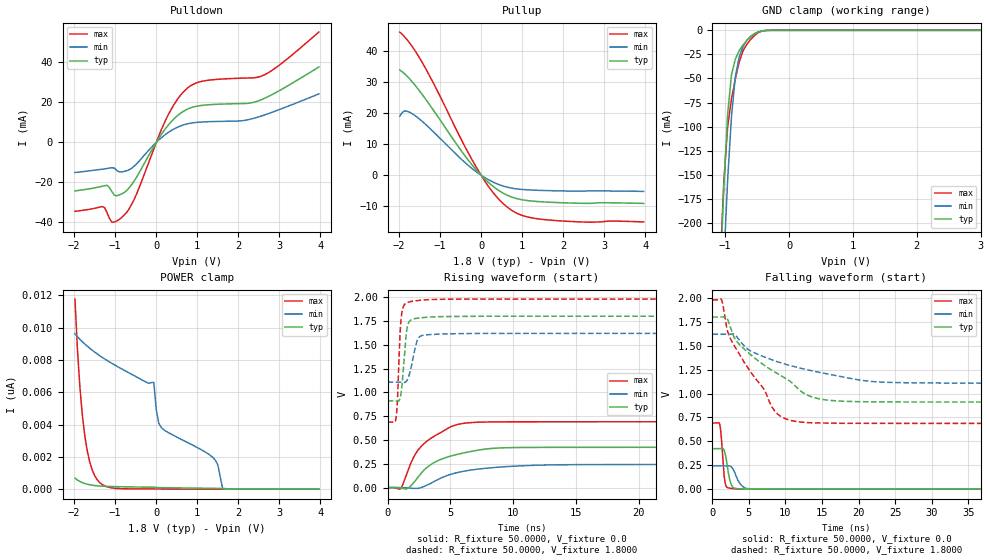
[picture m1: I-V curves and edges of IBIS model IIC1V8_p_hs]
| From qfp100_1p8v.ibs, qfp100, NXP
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[Model] IIC1V8_p_hs
|   Model IIC1V8_p_hs
| This model was characterised for following simulation conditions:
| External (pad) voltage:
|   - Typ: 1.8V,   - Min: 1.62V,   - Max: 1.98V
| Library cells for typ/min/max conditions are connected as defined below:
|  IO - External Pad
|  A - Core Input
|  EN - Output Buffer Enable
|  BOOST - vdde
|  EGP - vdd
|  EHS - vdd
|  ENZI - vdd
|  EPD - gnd
|  EPUN - vdd
|  ZI - NC
|  ZIF - NC
|  gnd - gnd
|  gnde - gnde
|  vdd - vdd
|  vdde - vdde
| All other pins connected to ground
Model_type I/O
Polarity   Non-Inverting
Enable   Active-Low
Vinl =   0.5400V
Vinh =   1.2600V
Vmeas =  0.9000V
Cref =   0.0F
Rref =   1.0000k
Vref =   0.0V
C_comp   3.6452pF   3.5037pF   3.7805pF
|C_comp_pullup   0.9522pF   0.9264pF   0.9623pF
|C_comp_pulldown   2.3410pF   2.4925pF   2.1970pF
[Model Spec]
| variable   typ   min   max
Vinh   0.5400V   0.4860V   0.5940V
Vinl   1.2600V   1.1340V   1.3860V
Vmeas   0.9000V   0.8100V   0.9900V
[Temperature Range]   25.0000   0.1250k   -40.0000
[Voltage Range]   1.8000V   1.6200V   1.9800V
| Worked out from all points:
|   slope of the pulldown table from 0 to 0.27 V, typ, clamps not added: 33.4 ohm
|   slope of the pullup table from 0 to 0.27 V, typ, clamps not added: 80.7 ohm
|   GND clamp passes 1 mA (typ) near -0.44 V on its own axis
|   rising waveform, R_fixture 50.0000, V_fixture 0.0: 20-80 % time 2.95ns typ, 3.71ns min, 2.38ns max; typ from 0 V to 0.423 V
|   rising waveform, R_fixture 50.0000, V_fixture 1.8000: 20-80 % time 334ps typ, 515ps min, 244ps max; typ from 0.911 V to 1.8 V
|   falling waveform, R_fixture 50.0000, V_fixture 0.0: 20-80 % time 582ps typ, 939ps min, 400ps max; typ from 0.423 V to 0 V
|   falling waveform, R_fixture 50.0000, V_fixture 1.8000: 20-80 % time 8.42ns typ, 11.2ns min, 5.75ns max; typ from 1.8 V to 0.911 V
[Pulldown]
|Voltage   I(typ)   I(min)   I(max)
-1.98V    -24.22mA   -15.04mA   -34.42mA
-1.32V    -21.94mA   -13.41mA   -32.06mA
-1.2V     -21.45mA   -13.05mA   -35.06mA
-1.08V    -24.63mA   -12.6mA    -39.9mA
-900mV    -26.23mA   -14.78mA   -38.53mA
-720mV    -24.07mA   -14.13mA   -34.99mA
-540mV    -19.33mA   -11.9mA    -28.53mA
300mV     8.856mA    5.096mA    14.12mA
720mV     16.26mA    9.117mA    26.48mA
1.14V     18.6mA     10.26mA    30.69mA
2.58V     21.56mA    13.35mA    33.32mA
3.96V     37.73mA    24.28mA    55.2mA
[Pullup]
|Voltage   I(typ)   I(min)   I(max)
-1.98V    33.84mA    18.97mA    46mA
-1.86V    32.57mA    20.67mA    44.44mA
-1.62V    29.12mA    19.27mA    40.26mA
-1.2V     21.64mA    14.46mA    30.6mA
-420mV    6.732mA    4.415mA    9.888mA
0V        251.1fA    74.01pA    -178.6fA
360mV     -4.265mA   -2.608mA   -6.666mA
660mV     -6.57mA    -3.917mA   -10.5mA
1.02V     -7.945mA   -4.606mA   -13.01mA
1.56V     -8.618mA   -4.934mA   -14.29mA
2.64V     -9.058mA   -5.064mA   -15.11mA
3.96V     -9.081mA   -5.209mA   -15.04mA
[GND_clamp]
|Voltage   I(typ)   I(min)   I(max)
-1.98V    -2.104A    -2.075A    -2.136A
-1.08V    -259.3mA   -333mA     -246.9mA
-1.02V    -161.8mA   -238.7mA   -157.1mA
-960mV    -86.74mA   -154.7mA   -99.46mA
-900mV    -45.95mA   -88.82mA   -71.05mA
-840mV    -29.9mA    -47.99mA   -50.25mA
-780mV    -21.15mA   -27.64mA   -32.98mA
-720mV    -15.16mA   -16.87mA   -21.26mA
-660mV    -10.56mA   -10.24mA   -14.56mA
-540mV    -3.788mA   -3.398mA   -5.292mA
-300mV    -15.94uA   -36uA      -16.34uA
3.96V     0A         0A         0A
[POWER_clamp]
|Voltage   I(typ)   I(min)   I(max)
-1.98V    679.6pA    9.61nA     11.76nA
-1.86V    475.2pA    9.277nA    6.313nA
-1.74V    349.2pA    8.982nA    3.292nA
-1.56V    245.6pA    8.597nA    1.186nA
-1.32V    186pA      8.161nA    293.2pA
-60mV     124.8pA    6.606nA    14.31pA
0V        105.5pA    4.916nA    11.81pA
120mV     93.21pA    3.82nA     10.91pA
1.38V     50pA       1.96nA     2.877pA
1.5V      45.28pA    1.501nA    2.149pA
1.62V     39.18pA    0A         1.42pA
3.96V     0A         0A         0A
[Ramp]
| variable   typ   min   max
dV/dt_r  0.2539/2.9459n   0.1457/3.7082n   0.4150/2.3771n
dV/dt_f  0.5334/8.4174n   0.3066/11.2444n   0.7753/5.7459n
R_load = 50.0000
[Rising Waveform]
R_fixture= 50.0000
V_fixture= 0.0
V_fixture_min= 0.0
V_fixture_max= 0.0
|time   V(typ)   V(min)   V(max)
0s        602.8pV    52.95nV    41.9pV
1.025ns   -3.559mV   224.6uV    -13.37mV
1.609ns   -8.623mV   -2.295mV   173.9mV
2.41ns    107mV      -7.915mV   390.7mV
3.322ns   231.1mV    37.35mV    506.5mV
4.754ns   320.6mV    127.8mV    619.6mV
6.036ns   363.4mV    171.4mV    674.9mV
9.05ns    417.3mV    216.6mV    690.6mV
24.7ns    423.2mV    242.7mV    691.6mV
1us       423.2mV    242.8mV    691.7mV
[Rising Waveform]
R_fixture= 50.0000
V_fixture= 1.8000
V_fixture_min= 1.6200
V_fixture_max= 1.9800
|time   V(typ)   V(min)   V(max)
0s        911mV      1.109V     687.8mV
690.7ps   908.9mV    1.109V     743.7mV
788.9ps   905.9mV    1.109V     924mV
1.019ns   951.7mV    1.108V     1.68V
1.284ns   1.297V     1.103V     1.909V
1.513ns   1.643V     1.119V     1.941V
1.772ns   1.751V     1.206V     1.952V
2.534ns   1.782V     1.583V     1.967V
4.752ns   1.797V     1.615V     1.978V
1us       1.8V       1.62V      1.98V
[Falling Waveform]
R_fixture= 50.0000
V_fixture= 0.0
V_fixture_min= 0.0
V_fixture_max= 0.0
|time   V(typ)   V(min)   V(max)
0s        423.2mV    242.8mV    691.7mV
1.027ns   423.3mV    242.8mV    673mV
1.231ns   425.9mV    242.8mV    537.8mV
1.605ns   407.6mV    242.8mV    144.1mV
1.873ns   326.1mV    244.3mV    32.56mV
2.289ns   128.2mV    244.4mV    11.82mV
2.696ns   32.02mV    224.4mV    6.498mV
3.717ns   3.925mV    64.61mV    1.806mV
4.701ns   1.508mV    7.232mV    669.6uV
1us       17.22nV    82.09nV    9.94nV
[Falling Waveform]
R_fixture= 50.0000
V_fixture= 1.8000
V_fixture_min= 1.6200
V_fixture_max= 1.9800
|time   V(typ)   V(min)   V(max)
0s        1.8V       1.62V      1.98V
1.239ns   1.8V       1.62V      1.984V
1.93ns    1.799V     1.62V      1.702V
2.441ns   1.7V       1.622V     1.579V
3.741ns   1.51V      1.552V     1.404V
8.553ns   1.224V     1.342V     815.3mV
10.66ns   1.127V     1.292V     720.4mV
15.13ns   938mV      1.215V     690.6mV
35.93ns   911.4mV    1.11V      688mV
1us       911mV      1.109V     687.8mV
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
